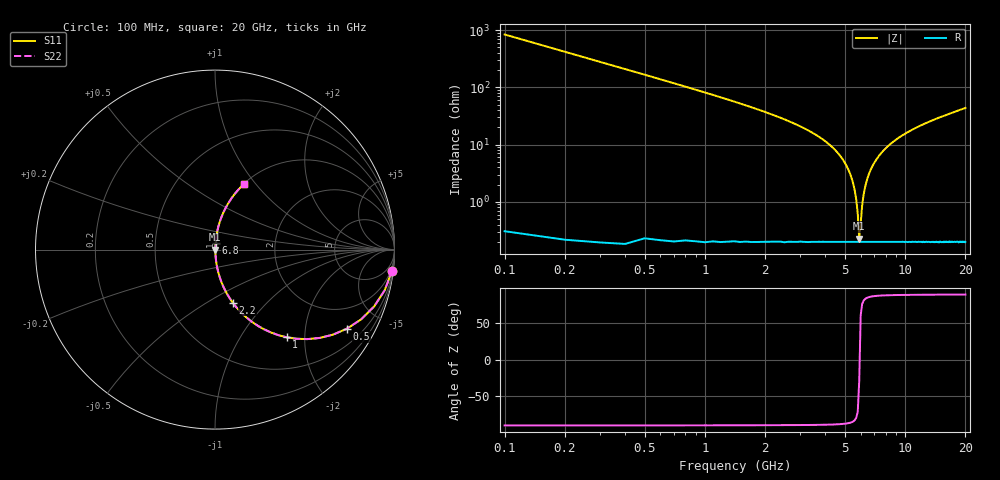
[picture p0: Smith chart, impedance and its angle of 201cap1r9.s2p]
! AVX Thin Film Operation		Date: May 2007
! Description: Accu-P® Series, Thin Film, SMD, RF Capacitor
! Part Number: 02013J1R9ABS
! 50 MHz  -  20.05 GHz
! Serial Measurements
# hz S db R 50
!	S11		S21		S12		S22
!	dB	Phase	dB	Phase	dB	Phase	dB	Phase
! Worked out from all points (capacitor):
!   200 points, 100 MHz to 20 GHz, reference 50 ohm
!   read as one part in series: C = 1.9 pF near 200 MHz
!   lowest |Z| = 229 mohm at 5.9 GHz (marker M1)
!   series resonance near 5.923 GHz, so ESL is about 380 pH
!   S11 on the Smith chart (normalised r, x): 100 MHz: 1, -17; 500 MHz: 1.00, -3.33; 1 GHz: 1.00, -1.63; 2.2 GHz: 1.00, -0.66; 6.8 GHz: 1.00, +0.08; 20 GHz: 1.00, +0.87
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1e8  -0.06 -6.8  -18.52 83.2  -18.52 83.2  -0.06 -6.8
2e8  -0.24 -13.4  -12.67 76.5  -12.67 76.5  -0.24 -13.4
3e8  -0.53 -19.8  -9.43 70.2  -9.43 70.2  -0.53 -19.8
5e8  -1.34 -31.0  -5.76 58.9  -5.76 58.9  -1.34 -31.0
1e9  -4.01 -50.8  -2.22 39.1  -2.22 39.1  -4.01 -50.8
1.5e9  -6.70 -62.2  -1.06 27.6  -1.06 27.6  -6.70 -62.2
2.2e9  -10.14 -71.5  -0.46 18.1  -0.46 18.1  -10.14 -71.5
3.5e9  -16.27 -80.4  -0.12 8.8  -0.12 8.8  -16.27 -80.4
4.6e9  -22.86 -84.3  -0.04 4.1  -0.04 4.1  -22.86 -84.3
5.3e9  -30.04 -84.6  -0.02 1.8  -0.02 1.8  -30.04 -84.6
5.7e9  -39.15 -78.9  -0.02 0.6  -0.02 0.6  -39.15 -78.9
5.8e9  -44.07 -71.0  -0.02 0.3  -0.02 0.3  -44.07 -71.0
5.9e9  -52.83 -28.9  -0.02 0.1  -0.02 0.1  -52.83 -28.9
6.1e9  -41.37 76.0  -0.02 -0.5  -0.02 -0.5  -41.37 76.0
6.2e9  -37.69 80.5  -0.02 -0.7  -0.02 -0.7  -37.69 80.5
6.4e9  -33.17 83.5  -0.02 -1.3  -0.02 -1.3  -33.17 83.5
6.8e9  -28.15 84.8  -0.02 -2.2  -0.02 -2.2  -28.15 84.8
8e9  -21.33 83.8  -0.05 -4.9  -0.05 -4.9  -21.33 83.8
1.01e10  -16.14 80.3  -0.12 -9.0  -0.12 -9.0  -16.14 80.3
1.34e10  -12.08 75.2  -0.29 -14.4  -0.29 -14.4  -12.08 75.2
1.67e10  -9.67 70.5  -0.51 -19.2  -0.51 -19.2  -9.67 70.5
2e10  -7.99 66.2  -0.77 -23.5  -0.77 -23.5  -7.99 66.2
